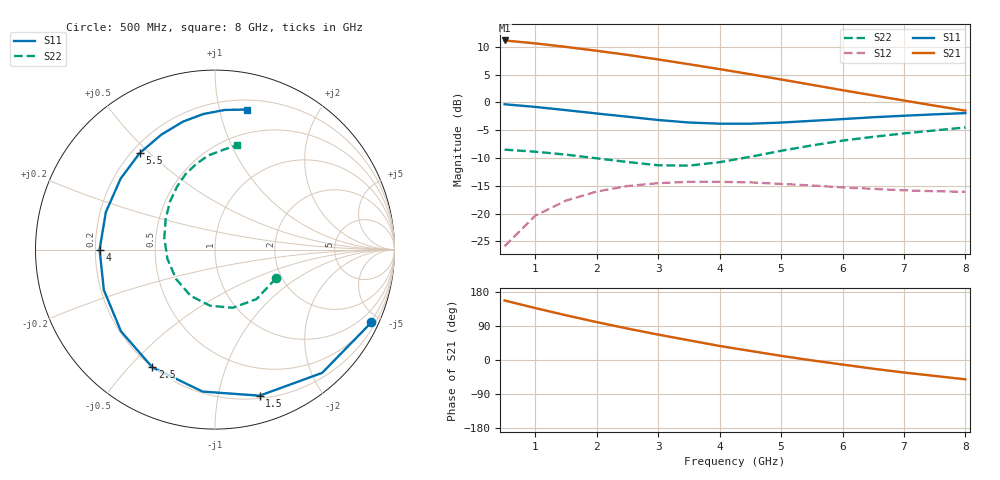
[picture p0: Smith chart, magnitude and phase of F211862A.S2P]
!ATF-21186
!S-PARAMETERS at Vds=2V  Id=10mA.  LAST UPDATED 01-30-98
# ghz s ma r 50
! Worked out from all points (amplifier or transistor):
!   16 points, 500 MHz to 8 GHz, reference 50 ohm
!   highest |S21| = 11.1 dB at 500 MHz (marker M1)
!   |S21| within 3 dB of that: start of sweep to 2.748 GHz
!   unconditionally stable (mu >= 1): 6.046 GHz to end of sweep
!   at 1.5 GHz: K = 0.33, MSG = 13.8 dB, |S12| = -17.7 dB
!   at 4.5 GHz: K = 0.83, MSG = 9.7 dB, |S12| = -14.4 dB
!   at 8 GHz: K = 1.08, MAG = 5.6 dB, |S12| = -16.1 dB
!   lowest NFmin = 0.37 dB at 500 MHz
!   S11 on the Smith chart (normalised r, x): 500 MHz: 0.42, -4.47; 1.5 GHz: 0.22, -1.33; 2.5 GHz: 0.20, -0.58; 4 GHz: 0.22, +0.00; 5.5 GHz: 0.23, +0.47; 8 GHz: 0.28, +1.22
0.5  0.961 -25.0  3.599 157.0  0.051 71.0  0.376 -25.0
1  0.91 -49.0  3.388 137.0  0.096 57.0  0.36 -50.0
1.5  0.851 -73.0  3.149 118.0  0.131 43.0  0.339 -73.0
2  0.794 -95.0  2.906 100.0  0.158 31.0  0.314 -95.0
2.5  0.743 -118.0  2.671 83.0  0.177 19.0  0.291 -118.0
3  0.694 -139.0  2.429 67.0  0.188 9.0  0.272 -143.0
3.5  0.659 -160.0  2.201 52.0  0.193 -1.0  0.27 -169.0
4  0.643 180.0  1.989 37.0  0.193 -9.0  0.29 167.0
4.5  0.643 161.0  1.789 24.0  0.191 -17.0  0.324 148.0
5  0.658 143.0  1.606 11.0  0.185 -24.0  0.367 133.0
5.5  0.682 128.0  1.438 -1.0  0.179 -29.0  0.41 121.0
6  0.707 115.0  1.286 -12.0  0.172 -34.0  0.453 111.0
6.5  0.735 104.0  1.155 -23.0  0.167 -38.0  0.49 102.0
7  0.758 95.0  1.038 -33.0  0.162 -41.0  0.526 94.0
7.5  0.78 86.0  0.934 -42.0  0.159 -44.0  0.559 85.0
8  0.801 77.0  0.842 -51.0  0.157 -47.0  0.595 78.0
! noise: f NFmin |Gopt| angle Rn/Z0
0.5  0.37  0.95  11  1.738
1  0.41  0.89  25  0.819
2  0.49  0.79  60  0.387
3  0.57  0.71  100  0.179
3.5  0.61  0.68  120  0.111
4.5  0.69  0.64  162  0.028
5.5  0.77  0.68  -155  0.042
6  0.81  0.73  -139  0.095
7  0.89  0.81  -111  0.362
8  0.97  0.86  -88  0.873
